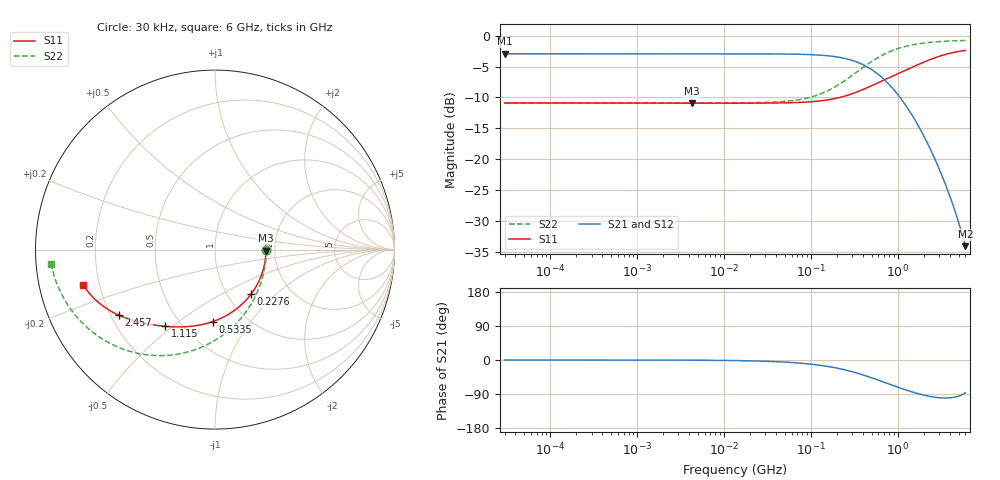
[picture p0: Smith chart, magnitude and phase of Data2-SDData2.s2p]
!EMIF06-MSD04F3
!Simulation
!24/03/11  09:23
!Start Freq. :30.000kHz; Stop Freq. : 6.000GHz
!Number of points : 1592; Sweep : LOGARITHMIC
!D2-D3 (Data2-SDData2)
!Freq ReS11 ImS11 ReS21 ImS21 ReS12 ImS12 ReS22 ImS22
# Hz  S  RI  R  50
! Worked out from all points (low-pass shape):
!   1592 points, 30 kHz to 6 GHz, reference 50 ohm
!   highest |S21| = -2.92 dB at 30 kHz (marker M1); lowest = -34.1 dB at 6 GHz (marker M2)
!   |S21| within 3 dB of the highest: start of sweep to 555.6 MHz
!   lowest |S11| = -10.9 dB at 4.27 MHz (marker M3), VSWR 1.79, Z = 89.7 - j1.04 ohm
!   |S11| at or under -10 dB: start of sweep to 214.9 MHz
!   |S22| runs from -10.9 to -0.8 dB; largest |S21 - S12| = 2e-15
!   S11 on the Smith chart (normalised r, x): 30 kHz: 1.80, -0.00; 227.6 MHz: 1.28, -0.71; 533.5 MHz: 0.71, -0.68; 1.115 GHz: 0.41, -0.47; 2.457 GHz: 0.23, -0.29; 6 GHz: 0.14, -0.13
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30000  0.2855 -0.000524  0.7142 -0.000312  0.7142 -0.000312  0.2857 -0.00021
231093.6  0.2844 -0.000787  0.7135 -0.000597  0.7135 -0.000597  0.2853 -0.000617
1766531  0.2841 -0.00231  0.7134 -0.00251  0.7134 -0.00251  0.2852 -0.00357
4270263  0.284 -0.00533  0.7133 -0.00592  0.7133 -0.00592  0.2852 -0.00856
1.350376e7  0.2837 -0.0166  0.7129 -0.0186  0.7129 -0.0186  0.2846 -0.027
4.336319e7  0.2806 -0.0531  0.7088 -0.0594  0.7088 -0.0594  0.2789 -0.0862
6.820056e7  0.2756 -0.083  0.7023 -0.0926  0.7023 -0.0926  0.2697 -0.1345
1.032257e8  0.265 -0.1238  0.6884 -0.1377  0.6884 -0.1377  0.2502 -0.2002
1.586553e8  0.2406 -0.1839  0.6567 -0.203  0.6567 -0.203  0.2058 -0.2957
2.275733e8  0.2004 -0.2489  0.6046 -0.2709  0.6046 -0.2709  0.1327 -0.3959
3.418125e8  0.1205 -0.3297  0.5027 -0.3471  0.5027 -0.3471  -0.0107 -0.5117
4.336319e8  0.0541 -0.3724  0.42 -0.3785  0.42 -0.3785  -0.1278 -0.5632
5.334838e8  -0.0137 -0.4015  0.3381 -0.39  0.3381 -0.39  -0.2446 -0.5876
6.463304e8  -0.0818 -0.4197  0.26 -0.3843  0.26 -0.3843  -0.3575 -0.5887
7.890804e8  -0.1544 -0.4292  0.183 -0.3618  0.183 -0.3618  -0.471 -0.5679
1.114606e9  -0.2768 -0.4277  0.0762 -0.2924  0.0762 -0.2924  -0.6378 -0.4914
1.611095e9  -0.4007 -0.4091  0.0103 -0.2026  0.0103 -0.2026  -0.7612 -0.3849
2.45728e9  -0.5354 -0.3659  -0.014 -0.1137  -0.014 -0.1137  -0.8444 -0.2676
3.117367e9  -0.6037 -0.3286  -0.0135 -0.077  -0.0135 -0.077  -0.8728 -0.2097
3.924532e9  -0.6603 -0.285  -0.0089 -0.0507  -0.0089 -0.0507  -0.8917 -0.1597
4.718326e9  -0.6973 -0.2468  -0.00435 -0.0351  -0.00435 -0.0351  -0.9023 -0.1234
6e9  -0.7345 -0.1958  0.00127 -0.0197  0.00127 -0.0197  -0.9117 -0.0801
